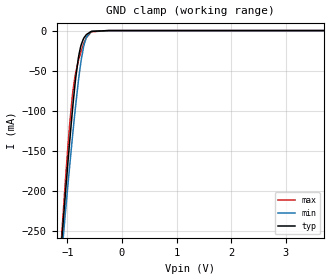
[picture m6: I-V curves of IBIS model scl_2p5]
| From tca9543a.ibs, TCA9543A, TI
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|   scl_2p5 Model
[Model]   scl_2p5
Model_type   Input
Vinl = 0.75
Vinh = 1.75
|   typ   min   max
|   (nom PVT)   (fast PVT)   (slow PVT)
C_comp   4.294e-12   3.611e-12   9.427e-12
[Model spec]
|subparameter
Vinl   0.75   0.675   0.825
Vinh   1.75   1.575   1.925
| Where nom  PVT is Nominal Process, 2.5V, 27C
|   Fast PVT is Strong Process,  2.75V, -40C
|   Slow PVT is Weak Process,   2.25V, 85C
[Voltage Range]   2.5   2.25   2.75
|Junction Temperature
[Temperature Range]   27   85   -40
[Power Clamp Reference]   2.5   2.25   2.75
[GND Clamp Reference]   0   0   0
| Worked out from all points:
|   GND clamp passes 1 mA (typ) near -0.55 V on its own axis
[GND Clamp]
|   Voltage   I(typ)   I(min)   I(max)
-2.5V     -1.62A     -1.464A    -1.842A
-1.109V   -266.3mA   -282.7mA   -259.5mA
-1.095V   -253.4mA   -271.4mA   -244.7mA
-1.034V   -200.7mA   -224.9mA   -184.2mA
-960mV    -139.1mA   -169.7mA   -117.6mA
-910.5mV  -100.9mA   -134.5mA   -81.91mA
-861mV    -66.92mA   -100.9mA   -57.25mA
-786.7mV  -29.33mA   -56.17mA   -34.51mA
-710mV    -10.86mA   -22.39mA   -17.7mA
-652.5mV  -5.003mA   -8.483mA   -8.825mA
-570mV    -1.34mA    -1.418mA   -2.165mA
5V        0A         0A         0A
[POWER Clamp]
|   Voltage   I(typ)   I(min)   I(max)
-2.5V     0A         0A         0A
-2.282V   0A         0A         0A
5V        0A         0A         0A
